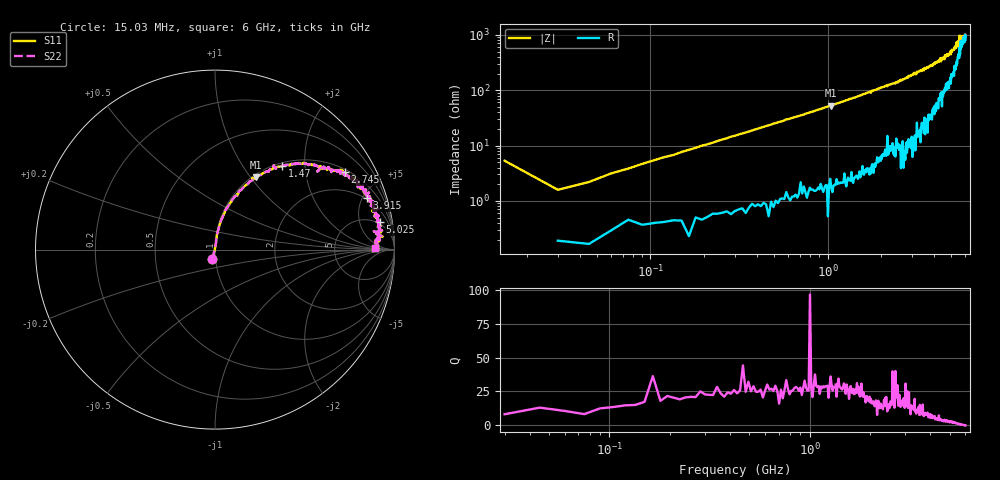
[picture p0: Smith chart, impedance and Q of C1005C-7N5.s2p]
!	Network	Analyzer	HP8753E.07.74:	Oct	30	2002	Serial	No.	JP38451487
!	Hewlett-Packard
!	7	Sep	2009	8:34:30
!	Frequency	S11	S21	S12	S22
#	HZ	S	RI	R	50
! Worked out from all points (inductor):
!   400 points, 15.03 MHz to 6 GHz, reference 50 ohm
!   read as one part in series: L = 8.08 nH near 45.03 MHz
!   highest Q = 29.1 at 1.05 GHz (marker M1), where L = 8.01 nH
!   S11 on the Smith chart (normalised r, x): 15.03 MHz: 0.97, -0.10; 1.47 GHz: 1.05, +1.54; 2.745 GHz: 1.11, +3.28; 3.915 GHz: 1.89, +5.43; 5.025 GHz: 4, +10; 6 GHz: 17, +1
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1.502992e7  -0.0148 -0.0524  1.01 0.0524  1.01 0.0524  -0.0148 -0.0524
3.002985e7  0.0023 0.0157  0.998 -0.0157  0.998 -0.0157  0.0023 0.0157
6.00297e7  0.00376 0.031  0.996 -0.031  0.996 -0.031  0.00376 0.031
1.200294e8  0.00781 0.061  0.992 -0.061  0.992 -0.061  0.00781 0.061
2.850286e8  0.0257 0.14  0.974 -0.14  0.974 -0.14  0.0257 0.14
5.850271e8  0.0923 0.266  0.908 -0.266  0.908 -0.266  0.0923 0.266
1.020025e9  0.218 0.395  0.782 -0.395  0.782 -0.395  0.218 0.395
1.050025e9  0.226 0.402  0.774 -0.402  0.774 -0.402  0.226 0.402
1.470023e9  0.376 0.467  0.624 -0.467  0.624 -0.467  0.376 0.467
2.01002e9  0.551 0.469  0.449 -0.469  0.449 -0.469  0.551 0.469
2.745016e9  0.723 0.431  0.277 -0.431  0.277 -0.431  0.723 0.431
3.015015e9  0.779 0.399  0.221 -0.399  0.221 -0.399  0.779 0.399
3.91501e9  0.847 0.287  0.153 -0.287  0.153 -0.287  0.847 0.287
4.00501e9  0.881 0.27  0.119 -0.27  0.119 -0.27  0.881 0.27
5.010005e9  0.907 0.161  0.0927 -0.161  0.0927 -0.161  0.907 0.161
5.025005e9  0.918 0.152  0.0816 -0.152  0.0816 -0.152  0.918 0.152
5.445003e9  0.925 0.0951  0.0752 -0.0951  0.0752 -0.0951  0.925 0.0951
5.535002e9  0.885 0.103  0.115 -0.103  0.115 -0.103  0.885 0.103
5.565002e9  0.935 0.0719  0.0648 -0.0719  0.0648 -0.0719  0.935 0.0719
5.595002e9  0.898 0.0909  0.102 -0.0909  0.102 -0.0909  0.898 0.0909
5.625002e9  0.919 0.0526  0.0808 -0.0526  0.0808 -0.0526  0.919 0.0526
6e9  0.891 0.00769  0.109 -0.00769  0.109 -0.00769  0.891 0.00769
